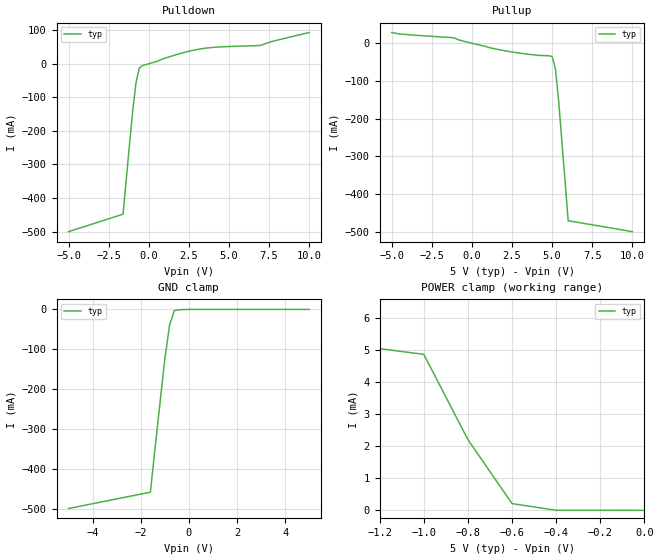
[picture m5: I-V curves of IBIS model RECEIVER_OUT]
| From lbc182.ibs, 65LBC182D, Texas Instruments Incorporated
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|   with 54ohm line-to-line and a 10pF cap from each
|   line-to-ground.
|   Receiver Output  MODEL
[Model]   RECEIVER_OUT
Model_type   3-state
| Signals   R
Vmeas = 2.0V   |Reference voltage for timing measurements
Cref = 15pF   |Timing specification test load capacitance value
Vref = 0   |Timing specification test load voltage; GND
| variable   typ   min   max
C_comp   1.0pF   NA   NA
|   typ   min   max
[Temperature Range]   25.0   NA   NA
[Voltage range]   5.0V   4.75V   5.25V
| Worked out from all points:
|   slope of the pulldown table from 0 to 0.75 V, typ, clamps not added: 62.3 ohm
|   slope of the pullup table from 0 to 0.75 V, typ, clamps not added: 101 ohm
|   GND clamp passes 1 mA (typ) near -0.40 V on its own axis
|   POWER clamp passes 1 mA (typ) near -0.68 V on its own axis
[Pulldown]
|   Voltage   I(typ)   I(min)   I(max)
-5V       -500mA     NA         NA
-1.6V     -448mA     NA         NA
-1V       -140mA     NA         NA
-800mV    -57.9mA    NA         NA
-600mV    -14mA      NA         NA
-400mV    -5.44mA    NA         NA
1.8V      28.4mA     NA         NA
3V        42.3mA     NA         NA
4.2V      49.4mA     NA         NA
7V        55mA       NA         NA
7.6V      65.4mA     NA         NA
10V       93mA       NA         NA
[Pullup]
|   Voltage   I(typ)   I(min)   I(max)
| Note that the[Pullup]voltage table is referenced to Vcc
| and is calculated using Vtable=Vcc - Vmeasured.
-5V       28.5mA     NA         NA
-4.4V     24.2mA     NA         NA
-1.2V     14.8mA     NA         NA
-600mV    6.38mA     NA         NA
1.8V      -17.9mA    NA         NA
3.4V      -28.5mA    NA         NA
5V        -35mA      NA         NA
5.2V      -66mA      NA         NA
5.4V      -150mA     NA         NA
6V        -471mA     NA         NA
10V       -500mA     NA         NA
[GND_clamp]
|   Voltage   I(typ)   I(min)   I(max)
| Outputs in High Impedance (off)
-5V       -500mA     NA         NA
-1.6V     -459mA     NA         NA
-1.4V     -346mA     NA         NA
-1.2V     -235mA     NA         NA
-1V       -125mA     NA         NA
-800mV    -38.5mA    NA         NA
-600mV    -2.67mA    NA         NA
-400mV    -988uA     NA         NA
-200mV    -467uA     NA         NA
0V        0A         NA         NA
5V        0A         NA         NA
[POWER_clamp]
|   Voltage   I(typ)   I(min)   I(max)
| Note that the [POWER_clamp] voltage table is referenced to Vcc
| and is calculated using Vtable = Vcc - Vmeasured.
| Outputs in Tri-state.
-5V       152mA      NA         NA
-4V       79.1mA     NA         NA
-3V       6.69mA     NA         NA
-2V       5.77mA     NA         NA
-1V       4.87mA     NA         NA
-800mV    2.21mA     NA         NA
-600mV    210uA      NA         NA
-400mV    3uA        NA         NA
0V        0A         NA         NA
[Ramp]
| Note: Ramp rate measured on single-ended Output.
|   typ   min   max
dV/dt_r   2.28/4.5ns   NA   NA
dV/dt_f   2.30/2.9ps   NA   NA
R_load = 50Ohm
